(* Logix 5000 Rung export; software revision 16.03 *)

MODULES
   PDPMV1_240 : vendor None type None code None
   Local : vendor None type None code None
END_MODULES

TYPE PDPMV1_SetSlaveMode_Out :   // Mailbox Request
STRUCT
   GroupSelect : SINT;   // Range 01h to FFh (Bit Coded). This parameter determines which group to address. Refer to the user manual for examples
   SlaveAddress : SINT;   // Range 1 to 125; 127 (Multicast address).
   ControlCommand : PDPMV1_ControlCommand;   // This parameter specifies the command to send (Unsync/Sync and Unfreeze/Freeze).
END_STRUCT
END_TYPE

TYPE PDPMV1_AbortConnection_In :
STRUCT
   C_REF : INT;   // Connection reference that shall be terminated.
   ReasonCode : SINT;   // Indicates the reason for the abort request. Value is user-specific. Range 0...15
   Subnet : SINT;   // This parameter encodes information about the origin of the abort initiator. 0: No 1: Local 2: Remote 3...255: (reserved)
   ExtendedFaultInformation : INT;   // If ‘Fault Information’ equals 000Ah or 000Bh, additional information of the error can be found here. For more information,
   FaultInformation : INT;   // If ‘Invalid Other’ is returned in the Message Information word in the header of the response,
END_STRUCT
END_TYPE

TYPE PDPMV1_SetSlaveMode_In :   // Mailbox response
STRUCT
   GroupSelect : SINT;   // Range 01h to FFh (Bit Coded). This parameter determines which group to address. Refer to the user manual for examples
   SlaveAddress : SINT;   // Range 1 to 125; 127 (Multicast address).
   ControlCommand : PDPMV1_ControlCommand;   // This parameter specifies the command to send (Unsync/Sync and Unfreeze/Freeze).
   ExtendedFaultInfo : INT;   // If other than 0, refer to user manual for code information
   FaultInformation : INT;   // If other than 0, refer to user manual for code information
END_STRUCT
END_TYPE

TYPE PDPMV1_Class2AcyclicRead_Out :
STRUCT
   C_REF : INT;   // Connection reference that shall be terminated
   Index : SINT;   // Used in the slave for addressing of the desired data block. Range 0...254
   SlotNumber : SINT;   // Used in the slave for addressing of the desired data block. Range 0...254
   Length : INT;   // Number of bytes to write
END_STRUCT
END_TYPE

TYPE PDPMV1_Class1AcyclicRead :   // DPV1 acyclic read mailbox data structure
STRUCT
   Out : PDPMV1_Class1AcyclicRead_Out;   // Mailbox request
   In : PDPMV1_Class1AcyclicRead_In;   // Mailbox response
END_STRUCT
END_TYPE

TYPE PDPMV1_Class1AcyclicRead_In :   // DPV1 acyclic read mailbox response
STRUCT
   ByteCount : INT;   // Byte count data block
   SlotNumber : SINT;   // Used in the slave to address the desired data block.
   SlaveAddress : SINT;   // Destination of slave (1-125)
   Length : SINT;   // Specifies the number of bytes of the data block to read
   Index : SINT;   // Index block
   ErrorDecode : SINT;   // If other than 0, refer to user manual for code information
   ErrorCode2 : SINT;   // If other than 0, refer to user manual for code information
   ErrorCode1 : SINT;   // If other than 0, refer to user manual for code information
   ExtendedFaultInfo : SINT;   // If other than 0, refer to user manual for code information
   FaultInformation : SINT;   // If other than 0, refer to user manual for code information
   Data : SINT[244];   // Returned data [1...n] array
END_STRUCT
END_TYPE

TYPE PDPMV1_AbortConnection :
STRUCT
   Out : PDPMV1_AbortConnection_out;   // Mailbox Request
   In : PDPMV1_AbortConnection_In;   // Mailbox Response
END_STRUCT
END_TYPE

TYPE PDPMV1_SetSlaveMode :   // SetSlaveMode mailbox that allows the processor to change the slave mode to interrupt input or output data update
STRUCT
   Out : PDPMV1_SetSlaveMode_Out;   // Mailbox Request
   In : PDPMV1_SetSlaveMode_In;   // Mailbox Response
END_STRUCT
END_TYPE

TYPE PDPMV1_GetSlaveConfig :   // GetSlaveConfig mailobox to retrieve configuration data from specific PROFIBUS slaves
STRUCT
   Out : PDPMV1_GetSlaveConfig_Out;   // mailbox request
   In : PDPMV1_GetSlaveConfig_In;   // mailbox response
END_STRUCT
END_TYPE

TYPE PDPMV1_other_status :
STRUCT
   Cfg_file_error : INT;   // Bit0 = PDPMV1.CFG, Bit 1 = WATTCP.CFG, Bit 2 = PDPMV1.DDB, Bit3=PDPMV1.XML
   R_120 : INT;   // Not Used
   R_122 : INT;   // Not Used
   R_124 : INT;   // Not Used
   R_126 : INT;   // Not Used
   R_128 : INT;   // Not Used
   R_130 : INT;   // Not Used
   R_132 : INT;   // Not Used
   R_134 : INT;   // Not Used
   R_136 : INT;   // Not Used
   R_138 : INT;   // Not Used
   R_140 : INT;   // Not Used
   R_142 : INT;   // Not Used
   R_144 : INT;   // Not Used
   In_MB_queue : INT;   // Number of messages in the input mailbox queue
   Out_MB_queue : INT;   // Number of messages in the output mailbox queue
   Alarm_MB_queue : INT;   // Number of messages in the alarm mailbox queue
   Last_out_MB : INT;   // Number of messages in the output mailbox queue
   Cur_in_MB : INT;   // Number of messages currently in the input mailbox queue
   Cur_alarm_MB : INT;   // Number of messages currently in the alarm mailbox queue
END_STRUCT
END_TYPE

TYPE PDPMV1_Class1AcyclicWrite_In :   // DPV1 acyclic write mailbox response
STRUCT
   ByteCount : INT;   // Byte count data block
   SlotNumber : SINT;   // Used in the slave to address the desired data block.
   SlaveAddress : SINT;   // Destination of slave (1-125)
   Length : SINT;   // Specifies the number of bytes of the data block to read
   Index : SINT;   // Index block
   ErrorDecode : SINT;   // If other than 0, refer to user manual for code information
   ErrorCode2 : SINT;   // If other than 0, refer to user manual for code information
   ErrorCode1 : SINT;   // If other than 0, refer to user manual for code information
   ExtendedFaultInfo : SINT;   // If other than 0, refer to user manual for code information
   FaultInformation : SINT;   // If other than 0, refer to user manual for code information
   Data : SINT[244];   // Returned data [1...n] array
END_STRUCT
END_TYPE

TYPE PDPMV1_Class2AcyclicWrite_Out :   // DPV1 acyclic write mailbox request
STRUCT
   DataSize : INT;   // Object data size
   C_REF : INT;   // Connection reference that shall be terminated
   Index : SINT;   // Index block
   SlotNumber : SINT;   // Used in the slave to address the desired data block.
   Length : INT;   // Specifies the number of bytes of the data block to read
   Data : SINT[244];   // Data that should be written [1...n]
END_STRUCT
END_TYPE

TYPE PDPMV1_SetSlaveAddress_In :   // Mailbox response
STRUCT
   ByteCount : INT;   // Byte count data block
   NewSlaveAddress : SINT;   // Range 1 to 125, specifies the new address of the slave
   CurrentSlaveAddress : SINT;   // Range 1 to 125, specifies the current address of the slave
   SlaveIdentNumber : INT;   // Indent number for the slave
   No_add_Chg : INT;   // specifies whether it is allowed to change the slave address again later
   ErrorCode1_2 : INT;   // If other than 0, refer to user manual for code information
   ErrorCode3_4 : INT;   // If other than 0, refer to user manual for code information
   ReturnCode : INT;   // If other than 0, refer to user manual for code information
   FaultInformation : INT;   // If other than 0, refer to user manual for code information
   MessageDataByte : SINT[400];   // Message data byte array for user-specific data
END_STRUCT
END_TYPE

TYPE PDPMV1_SetSlaveAddress_Out :   // Mailbox request
STRUCT
   ByteCount : INT;   // Byte count data block
   NewSlaveAddress : SINT;   // Range 1 to 125, specifies the new address of the slave
   CurrentSlaveAddress : SINT;   // Range 1 to 125, specifies the current address of the slave
   SlaveIdentNumber : INT;   // Indent number for the slave
   No_add_Chg : INT;   // specifies whether it is allowed to change the slave address again later
   MessageDataByte : SINT[400];   // Message data byte array for user-specific data
END_STRUCT
END_TYPE

TYPE PDPMV1_backplane :   // This object stores variables used by the sample ladder for handshaking.
STRUCT
   Read : INT;   // Backplane read statistics
   Write : INT;   // Backplane write statistics
   Error : INT;   // Backplane error statistics
   LastRead : INT;   // Last read block index received from the module
   LastWrite : INT;   // Last write block index received from the module
   BlockIndex : INT;   // Block index of each copy of PROFIBUS input and output blocks
END_STRUCT
END_TYPE

TYPE PDPMV1_GetSlaveDiagnostics_In :   // GetSlaveDiagnostics mailbox response
STRUCT
   RequestType : SINT;   // Type of request. 0 to use module memory RAM or 1 for live PROFIBUS network.
   SlaveAddress : SINT;   // Destination of slave (Range 1-125)
   ExtendedFaultInfo : INT;   // If other than 0, refer to user manual for code information
   FaultInformation : INT;   // If other than 0, refer to user manual for code information
   StationStatus1_2 : INT;   // Status of station types 1 and 2
   StationStatus3_4 : INT;   // Status of station types 3 and 4
   IdentNumber : INT;   // Unique ID assigned by the PROFIBUS User Organization
   ExtendedDiagnosticData : INT[200];   // Slave user-specific data. Refer to actual slave documentation for info
END_STRUCT
END_TYPE

TYPE PDPMV1_ControlCommand :   // Option bits for SetSlaveMode mailbox
STRUCT
   Reserved1 : BOOL;   // Reserved
   Reserved2 : BOOL;   // Reserved
   Unfreeze_Input : BOOL;   // Freeze mode is concluded when initiated
   Freeze_Input : BOOL;   // Causes the addressed slave to assume freeze mode.
   Unsynchronize_Output : BOOL;   // Unsynchronized output data
   Synchronize_Output : BOOL;   // Synchronized output data
   Reserved3 : BOOL[32];   // Reserved
END_STRUCT
END_TYPE

TYPE PDPMV1_InitiateConnection_out :
STRUCT
   SlaveAddress : INT;   // Address of the slave to which a connection shall be established. Range: 0...126
   C_REF : INT;   // Connections references used to identify the connection later on. Range: 1-128
END_STRUCT
END_TYPE

TYPE PDPMV1_CRC :   // This object stores CRC values for both Profibus and the module.
STRUCT
   ProfibusCRC : DINT;   // Stores Profibus CRC32 values
   ModuleCRC : DINT;   // Stores Module CRC32 values
END_STRUCT
END_TYPE

TYPE PDPMV1_Fieldbus :   // Fieldbus status
STRUCT
   FB_Slave_Cfg_List : SINT[16];   // Bitmap structure containing PROFIBUS slave configuration (bit x = 1 means slave x is configured)
   FB_Slave_Data_xfer : SINT[16];   // Bitmap structure containing PROFIBUS slave data exchange status (bit x = 1 means slave x is transferring data to the module)
   FB_Slave_Diag : SINT[16];   // Bitmap structure containing PROFIBUS slave diagnostic info (bit x = 1 means slave x is reporting diagnostics)
   FB_Pad_Byte : SINT;   // Reserved
   FB_op_state : SINT;   // Operation state ( 00 = offline, 40 = stop, 80 = clear, C0= operate)
   FB_ident_MSB : SINT;   // Master identification code (most significant byte)
   FB_ident_LSB : SINT;   // Master identification code (least significant byte)
END_STRUCT
END_TYPE

TYPE PDPMV1_GetSlaveDiagnostics :   // GetSlaveDiagnostics mailbox to retrieve diagnostic information from specific PROFIBUS slaves
STRUCT
   Out : PDPMV1_GetSlaveDiagnostics_Out;   // Mailbox request
   In : PDPMV1_GetSlaveDiagnostics_In;   // Mailbox response
END_STRUCT
END_TYPE

TYPE PDPMV1_Class1AcyclicWrite_Out :   // DPV1 acyclic write mailbox request
STRUCT
   SlotNumber : SINT;   // Used in the slave to address the desired data block.
   SlaveAddress : SINT;   // Destination of slave (1-125)
   DataSize : INT;   // Object data size
   Length : SINT;   // Specifies the number of bytes of the data block to read
   Index : SINT;   // Index block
   Data : SINT[244];   // Data that should be written [1...n]
END_STRUCT
END_TYPE

TYPE PDPMV1_Module :   // Status data
STRUCT
   Mod_scan_count : INT;   // Incremented every module scan loop
   Mod_output_update : INT;   // Incremented at every output scan
   Mod_input_update : INT;   // Incremented at every input scan
   Mod_out_MB : INT;   // Incremented at every output mailbox processing
   Mod_in_MB : INT;   // Incremented at every intput mailbox processing
   Mod_alarm_ind : INT;   // Incremented at every alarm indication
   Mod_alarm_con : INT;   // Incremented at every alarm confirmation
   Reserved1 : INT;   // Reserved
   Reserved2 : INT;   // Reserved
END_STRUCT
END_TYPE

TYPE PDPMV1_Class1AcyclicRead_Out :   // DPV1 acyclic read mailbox request
STRUCT
   SlotNumber : SINT;   // Used in the slave to address the desired data block.
   SlaveAddress : SINT;   // Destination of slave (1-125)
   DataSize : INT;   // Object data size
   Length : SINT;   // Specifies the number of bytes of the data block to read
   Index : SINT;   // Index block
END_STRUCT
END_TYPE

TYPE PDPMV1_backplane2 :   // This object stores variables used by the sample ladder for handshaking.
STRUCT
   LastRead : INT;   // Last read block index received from the module
   LastWrite : INT;   // Last write block index received from the module
   BlockIndex : INT;   // Block index of each copy of PROFIBUS input and output blocks
END_STRUCT
END_TYPE

TYPE PDPMV1_Start_Stop_Slaves_In :   // Mailbox response
STRUCT
   AdditionalFaultInfo : INT;   // If other than 0, refer to user manual for code information
   FaultInformation : INT;   // If other than 0, refer to user manual for code information
   SlaveNumber : SINT[126];   // Slave number designation (1-125)
END_STRUCT
END_TYPE

TYPE PDPMV1_InitiateConnection :
STRUCT
   Out : PDPMV1_InitiateConnection_out;   // Mailbox Request
   In : PDPMV1_InitiateConnection_In;   // Mailbox response
END_STRUCT
END_TYPE

TYPE PDPMV1_Class2AcyclicRead_In :
STRUCT
   DataSize : INT;   // Byte count data block
   C_REF : INT;   // Connections references used to identify the connection later on. Range: 1-128
   Index : SINT;   // Index block
   SlotNumber : SINT;   // Used in the slave to address the desired data block.
   Length : INT;   // Specifies the number of bytes of the data block to read
   ErrorDecode : INT;   // If other than 0, refer to user manual for code information
   ErrorCode2 : SINT;   // If other than 0, refer to user manual for code information
   ErrorCode1 : SINT;   // If other than 0, refer to user manual for code information
   ExtendedFaultInfo : SINT;   // If other than 0, refer to user manual for code information
   FaultInformation : SINT;   // If other than 0, refer to user manual for code information
   Data : SINT[244];   // Returned data [1...n] array
END_STRUCT
END_TYPE

TYPE PDPMV1_Control :   // Control status
STRUCT
   serial_number : SINT[4];   // Module serial number
   version_MSB : SINT;   // Module version number (most significant byte)
   version_LSB : SINT;   // Module version number (least significant byte)
   mod_status_MSB : SINT;   // Module status (most significant byte)
   mod_status_LSB : SINT;   // Module status (least significant byte)
END_STRUCT
END_TYPE

TYPE PDPMV1_Command :   // This object contains the command bits that request mailbox messages from the module.
STRUCT
   StopMode : BOOL;   // Set the module to stop mode (PROFIBUS communication is interrupted in stop mode)
   OperateMode : BOOL;   // Set the module to operate mode (module only communicates through PROFIBUS)
   ClearMode : BOOL;   // Set the module to clear mode (outputs are disabled)
   SynchCRC : BOOL;   // CRC synchronization
   GetLiveList : BOOL;   // Request the Live List information from the module
   GetSlaveConfig : BOOL;   // Request configuration information from a slave
   SetSlaveMode : BOOL;   // Set the module to stop mode (PROFIBUS communication is interrupted in stop mode)
   GetSlaveDiagnostics : BOOL;   // Requests slave diagnostics from a slave
   SetSlaveAddress : BOOL;   // Change the slave's PROFIBUS address (only if slave supports this feature)
   StartSlaves : BOOL;   // Restarts PROFIBUS communication with one or more slaves after a "StopSlave" mailbox
   StopSlaves : BOOL;   // Stop PROFIBUS communication with one or more slaves
   Class1AcyclicRead : BOOL;   // Request the module to send acyclic read message to the slave
   Class1AcyclicWrite : BOOL;   // Request the module to send acyclic write message to slave
   InitiateConnection : BOOL;   // Request to establish connection with a V1 slave that can handle class 2 messages
   AbortConnection : BOOL;   // Request to Abort an already established connection with a V1 slave that can handle class 2 messages
   Class2AcyclicRead : BOOL;   // Request the module to send class 2 acyclic Read message to a V1 slave
   Class2AcyclicWrite : BOOL;   // Request the module to send class 2 acyclic Write message to a V1 slave
END_STRUCT
END_TYPE

TYPE PDPMV1_ModuleDef :   // Main module definition
STRUCT
   Output : SINT[1536];   // Output data
   Input : SINT[1536];   // Input data
   BP : PDPMV1_backplane2;   // Backplane status
   Status : PDPMV1_Status;   // Module status information
   MailboxCommand : PDPMV1_Command;   // Mailbox Command
   Mailbox : PDPMV1_Mailbox;   // Mailbox tags for optional applications
   CRC : PDPMV1_CRC_Struct;   // CRC status
   MailboxControl : PDPMV1_MBControl;   // Mailbox Control
   Util : PDPMV1_Util;   // Internal tags used for ladder logic processing. User applications should not overwrite any Util tags
END_STRUCT
END_TYPE

TYPE PDPMV1_GetSlaveConfig_Out :   // GetSlaveConfig mailbox request
STRUCT
   SlaveAddress : INT;   // Destination of slave (1-125)
END_STRUCT
END_TYPE

TYPE PDPMV1_GetSlaveDiagnostics_Out :   // GetSlaveDiagnostics mailbox request
STRUCT
   RequestType : SINT;   // Type of request. 0 to use module memory RAM or 1 for live PROFIBUS network.
   SlaveAddress : SINT;   // Destination of slave (Range 1-125)
END_STRUCT
END_TYPE

TYPE PDPMV1_Class1AcyclicWrite :   // DPV1 acyclic write mailbox data structure
STRUCT
   Out : PDPMV1_Class1AcyclicWrite_Out;   // Mailbox request
   In : PDPMV1_Class1AcyclicWrite_In;   // Mailbox response
END_STRUCT
END_TYPE

TYPE PDPMV1_InitiateConnection_In :   // This tag holds the response parameters after the user sends mailbox to initiate connection with V1 slave
STRUCT
   SizeofdatainBytes : INT;   // Size of data being read
   C_REF : INT;   // Connections references used to identify the connection later on. Range: 1-128
   MaxDataLength : SINT;   // The slave’s maximum data length in bytes (reported by the slave in DP Initiate.res).
   SlaveAddress : SINT;   // Address of the slave to which a connection shall be established. Range: 0...126
   MinmumSlaveTimeout : INT;   // The minimum slave timeout value supported by the slave (in multiples of 10ms).
   ErrorDecode : SINT;   // If ‘Fault Information’ equals 0010h, additional information according to the DPV1 specification
   ErrorCode2 : SINT;   // If ‘Fault Information’ equals 0010h, additional information according to the DPV1 specification
   ErrorCode1 : SINT;   // If ‘Fault Information’ equals 0010h, additional information according to the DPV1 specification
   ExtendedFaultInformation : INT;   // If ‘Fault Information’ equals 000Ah or 000Bh, additional information of the error can be found here. For more information, see
   FaultInformation : INT;   // If ‘Invalid Other’ is returned in the Message Information word in the header of the response, information about the fault
   SendTimeout : INT;   // Defines the control time (timebase 10ms) for the supervision of the connection between the slave and the master. Range 6...655
   FeatureSupported2 : SINT;   // (reserved for future use)
   FeatureSupported1 : SINT;   // Identifies the supported C2-service functionality as follows: b0: DPV1_RW. This bit is set if the services C2_Read and C2_Write
   ProfileFeatures2 : SINT;   // Identifies the supported service functionality regarding the used profile definition. The meaning of these registers are profil
   ProfileFeatures1 : SINT;   // Identifies the supported service functionality regarding the used profile definition. The meaning of these registers are profil
   ProfileIdentNumber : INT;   // This parameter identifies a unique profile definition. The Profile Ident Number is taken from the pool of Ident Numbers managed
   S_Length : SINT;   // This parameter specifies the length of the S_Address parameter (see table below). Default value is 02h.
   S_Type : SINT;   // This parameter indicates the presence of the optional Network/MAC address of the source. b0: 1: A Network/MAC address is presen
   D_Length : SINT;   // This value specifies the length of the D_Address parameter (see table below). Default value is 02h.
   D_Type : SINT;   // This parameter indicates the presence of the optional Network/MAC address of the destination. b0: 1: A Network/MAC address is p
   S_Address : INT;   // This field holds additional address information about the source. It’s structure depends on the settings in S_Type.
   D_Address : INT;   // This field holds additional address information about the destination. It’s structure depends on the settings in D_Type
END_STRUCT
END_TYPE

TYPE PDPMV1_Class2AcyclicWrite :   // DPV1 acyclic write mailbox data structure
STRUCT
   Out : PDPMV1_Class2AcyclicWrite_Out;   // Mailbox request
   In : PDPMV1_Class2AcyclicWrite_In;   // Mailbox response
END_STRUCT
END_TYPE

TYPE PDPMV1_GetLiveList :   // GetLiveList mailbox to retrieve the live list information from PROFIBUS network, informing the slaves that are communicating
STRUCT
   ReturnCode : SINT;   // Returned code about the nodes on the network
   FaultInfo : SINT;   // If other than 0, refer to user manual for code information
   Station : SINT[127];   // Station type contents.
END_STRUCT
END_TYPE

TYPE PDPMV1_AbortConnection_out :
STRUCT
   C_REF : INT;   // Connection reference that shall be terminated
   ReasonCode : SINT;   // Indicates the reason for the abort request. Value is user-specific. Range 0...15.
   Subnet : SINT;   // This parameter encodes information about the origin of the abort initiator. 0: No 1: Local 2: Remote
END_STRUCT
END_TYPE

TYPE PDPMV1_GetSlaveConfig_In :   // GetSlaveConfig mailbox response
STRUCT
   ByteCount : INT;   // Byte count data block
   WordCount : INT;   // Word count data block
   SlaveAddress : INT;   // Destination of slave (1-125)
   ErrorCode : INT[1];   // If other than 0, refer to user manual for code information
   ReturnCode : INT;   // If other than 0, refer to user manual for code information
   FaultInformation : INT;   // If other than 0, refer to user manual for code information
   Identifier : SINT[245];   // Configuration from a specific connected PROFIBUS slave
END_STRUCT
END_TYPE

TYPE PDPMV1_Util :
STRUCT
   ByteSwapUtil : INT;   // Used for byte swap logic
   TempInt : INT;   // Used for integer formatting
   UtilCount : INT;   // Used for util count range
END_STRUCT
END_TYPE

TYPE PDPMV1_CRC_Struct :   // Module CRC structures
STRUCT
   In : PDPMV1_CRC;   // Mailbox response
   Out : PDPMV1_CRC;   // Mailbox request
END_STRUCT
END_TYPE

TYPE PDPMV1_Class2AcyclicWrite_In :   // DPV1 acyclic write mailbox response
STRUCT
   ByteCount : INT;   // Byte count data block
   C_REF : INT;   // Connection reference that shall be Read
   Index : SINT;   // Index block
   SlotNumber : SINT;   // Used in the slave to address the desired data block.
   Length : SINT;   // Specifies the number of bytes of the data block to read
   ErrorDecode : SINT;   // If other than 0, refer to user manual for code information
   ErrorCode2 : SINT;   // If other than 0, refer to user manual for code information
   ErrorCode1 : SINT;   // If other than 0, refer to user manual for code information
   ExtendedFaultInfo : SINT;   // If other than 0, refer to user manual for code information
   FaultInformation : SINT;   // If other than 0, refer to user manual for code information
   Data : SINT[244];   // Returned data [1...n] array
END_STRUCT
END_TYPE

TYPE PDPMV1_MBControl :   // PDPMV1 MBControl status.
STRUCT
   Out_MB_index : INT;   // Reserved
   In_MB_index : INT;   // Reserved
   Alarm_MB_index : INT;   // Reserved
   In_Last_Out_MB : INT;   // Last out mailbox message ID processed from output image
   In_Last_In_MB : INT;   // Current in mailbox control index
   In_Last_Alarm_MB : INT;   // Current alarm control index
   Out_Last_Out_MB : INT;   // Reserved
   Out_Last_In_MB : INT;   // Reserved
   Out_Last_Alarm_MB : INT;   // Reserved
END_STRUCT
END_TYPE

TYPE PDPMV1_Start_Stop_Slaves_Out :   // Mailbox request
STRUCT
   SlaveNumber : SINT[126];   // Slave number designation (1-125)
END_STRUCT
END_TYPE

TYPE PDPMV1_Mailbox :   // Stores all mailbox request and response registers
STRUCT
   GetLiveList : PDPMV1_GetLiveList;   // Gets information from all nodes on the network
   GetSlaveConfig : PDPMV1_GetSlaveConfig;   // Get slave configuration
   SetSlaveMode : PDPMV1_SetSlaveMode;   // Send special control command to one or several slaves (Sync/Freeze)
   GetSlaveDiagnostics : PDPMV1_GetSlaveDiagnostics;   // Get diagnostic information from a slave
   SetSlaveAddress : PDPMV1_SetSlaveAddress;   // Set node address of a slave (if supported by the slave)
   StartStopSlaves : PDPMV1_Start_Stop_Slaves;   // Start/Stop slaves dynamically
   Class1AcyclicRead : PDPMV1_Class1AcyclicRead;   // Initiates a DPV1 class 1 acyclic read request.
   Class1AcyclicWrite : PDPMV1_Class1AcyclicWrite;   // Initiates a DPV1 class 1 acyclic write request.
   Alarm : PDPMV1_Alarm;   // Alarm message transferred by a slave to the master
   InitiateConnection : PDPMV1_InitiateConnection;   // mailbox form used to initiate connection with v1 slave before sending class2 messages.
   AbortConnection : PDPMV1_AbortConnection;   // mailbox form used to abort an already established connection with v1 slave before sending class2 messages.
   Class2AcyclicRead : PDPMV1_Class2AcyclicRead;   // mailbox form used to send a class 2 messages to read acyclic data
   Class2AcyclicWrite : PDPMV1_Class2AcyclicWrite;
END_STRUCT
END_TYPE

TYPE PDPMV1_Start_Stop_Slaves :   // Start/Stop Slaves mailbox allows the processor to restart or hault slave communication.
STRUCT
   Out : PDPMV1_Start_Stop_Slaves_Out;   // Mailbox Request
   In : PDPMV1_Start_Stop_Slaves_In;   // Mailbox Response
END_STRUCT
END_TYPE

TYPE PDPMV1_Alarm :   // DPV1 alarm data received by the module
STRUCT
   ByteCount : INT;   // Byte count data block
   SlotNumber : SINT;   // Used in the slave to address the desired data block. Range 0-254
   SlaveAddress : SINT;   // Destination of slave (1-125)
   AlarmSpecAck : SINT;   // Additional alarm information
   SeqNumber : SINT;   // Unique ID number of the alarm. Range 0-31.
   ExtDiag : SINT;   // Extended Diagnostic Flag (FFh - flag set and 00h - flag cleared).
   AlarmType : SINT;   // Identifies alarm type. Range is from 1 to 6, 32 to 126.
   FaultInformation : SINT;   // If other than 0, refer to user manual for code information
   Data : SINT[500];   // Returned data [1...n] array with additional manf. spec alarm info.
END_STRUCT
END_TYPE

TYPE PDPMV1_SetSlaveAddress :   // SetSlaveAddress mailbox that allows the module to dynamically change a PRIDUBUS address (only for slaves that supports it)
STRUCT
   Out : PDPMV1_SetSlaveAddress_Out;   // Mailbox request
   In : PDPMV1_SetSlaveAddress_In;   // Mailbox response
END_STRUCT
END_TYPE

TYPE PDPMV1_Class2AcyclicRead :
STRUCT
   Out : PDPMV1_Class2AcyclicRead_Out;   // Mailbox request
   In : PDPMV1_Class2AcyclicRead_In;   // Mailbox response
END_STRUCT
END_TYPE

TYPE PDPMV1_Status :   // Status block 0 or -1 for the MVI56-PDPMV1 module
STRUCT
   Pattern : SINT[12];   // Module indentification code
   Input_Size : INT;   // Input data size
   Output_Size : INT;   // Output data size
   Reserved_16 : INT;   // Reserved
   Reserved_18 : INT;   // Reserved
   Reserved_20 : INT;   // Reserved
   Input_Swap : SINT;   // User configured flag to indicate if input data is swapped before placing in the input image of the controller
   Output_Swap : SINT;   // User configured flag to indicate if output data is swapped before placing in the output image of the controller
   Module_Major_Ver : SINT;   // Module software major version number
   Module_Minor_Ver : SINT;   // Module software minor version number
   Fieldbus : PDPMV1_Fieldbus;   // PROFIBUS network status information
   Control : PDPMV1_Control;   // Module information
   Profibus_CRC32 : DINT;   // Profibus CRC32 value
   Module_CRC32 : DINT;   // Module CRC32 value
   Module : PDPMV1_Module;   // General module status to monitor data, mailbox and alarm exchange between the processor and the module
   Backplane : PDPMV1_backplane;   // Backplane status information
   Other : PDPMV1_other_status;   // General mailbox and cfg error information
END_STRUCT
END_TYPE

ADD_ON_INSTRUCTION AOI69PDPMV1_240   (* revision 1.4, vendor ProSoft Technology Inc. *)
// Add-On - MVI69-PDPMV1(Block size 240).
// Revision note:
// v1.4 - Added support for class 2 messages that was supported in a specific  V1 slaves.
VAR_IN_OUT
   Connection_Input : INT[242]; {required}   // Connection Input to be associated to the MVI69PDPMV1 Input Array
   Connection_Output : INT[241]; {required}   // Connection Output to be associated to the MVI69-PDPMV1 Output Array
   MVI69PDPMV1 : PDPMV1_ModuleDef; {required}
END_VAR

ROUTINE Logic   (* ladder *)
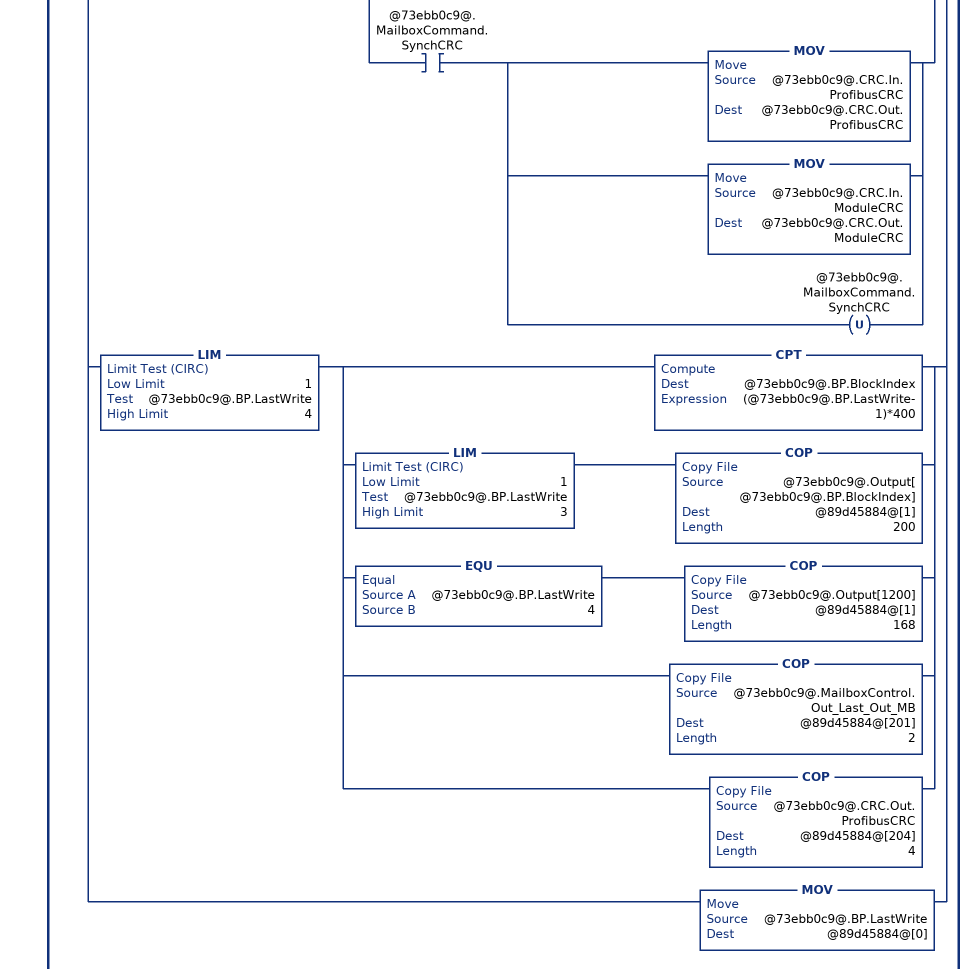
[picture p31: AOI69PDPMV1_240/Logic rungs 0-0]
   // This rung is used to verify if the module has sent a new input block to the processor. The trigger is when the input image offset 0 (Read Block ID) is different than the last one processed by the processor
   0: NEQ(@8034a877@[0],@73ebb0c9@.BP.LastRead)[MOV(@8034a877@[0],@73ebb0c9@.BP.LastRead) ,[EQU(@73ebb0c9@.BP.LastRead,-1) ,EQU(@73ebb0c9@.BP.LastRead,0) ] [COP(@8034a877@[2],@73ebb0c9@.Status.Pattern[0],20) ,COP(@8034a877@[13],@73ebb0c9@.Status.Input_Swap,4) ,COP(@8034a877@[15],@73ebb0c9@.Status.Fieldbus.FB_Slave_Cfg_List[0],52) ,COP(@8034a877@[41],@73ebb0c9@.Status.Control.serial_number[0],8) ,COP(@8034a877@[45],@73ebb0c9@.Status.Profibus_CRC32,2) ,COP(@8034a877@[49],@73ebb0c9@.Status.Module.Mod_scan_count,9) ,COP(@8034a877@[58],@73ebb0c9@.Status.Backplane.Read,3) ,COP(@8034a877@[61],@73ebb0c9@.Status.Other.Cfg_file_error,20) ] ,LIM(1,@73ebb0c9@.BP.LastRead,4) [LIM(1,@73ebb0c9@.BP.LastRead,3) [CPT(@73ebb0c9@.BP.BlockIndex,(@73ebb0c9@.BP.LastRead-1)*400) ,COP(@8034a877@[2],@73ebb0c9@.Input[@73ebb0c9@.BP.BlockIndex],400) ] ,EQU(@73ebb0c9@.BP.LastRead,4) COP(@8034a877@[2],@73ebb0c9@.Input[1200],336) ,COP(@8034a877@[202],@73ebb0c9@.MailboxControl.In_Last_Out_MB,2) ,COP(@8034a877@[206],@73ebb0c9@.CRC.In.ProfibusCRC,2) ] ,LIM(100,@73ebb0c9@.BP.LastRead,109) [LIM(0,@8034a877@[2],2) [OTU(@73ebb0c9@.MailboxCommand.StopMode) ,OTU(@73ebb0c9@.MailboxCommand.OperateMode) ,OTU(@73ebb0c9@.MailboxCommand.ClearMode) ,OTU(@73ebb0c9@.MailboxCommand.SynchCRC) ,OTU(@73ebb0c9@.MailboxCommand.GetLiveList) ,OTU(@73ebb0c9@.MailboxCommand.GetSlaveConfig) ,OTU(@73ebb0c9@.MailboxCommand.SetSlaveMode) ,OTU(@73ebb0c9@.MailboxCommand.GetSlaveDiagnostics) ,OTU(@73ebb0c9@.MailboxCommand.SetSlaveAddress) ,OTU(@73ebb0c9@.MailboxCommand.Class1AcyclicRead) ,OTU(@73ebb0c9@.MailboxCommand.Class1AcyclicWrite) ,OTU(@73ebb0c9@.MailboxCommand.StartSlaves) ,OTU(@73ebb0c9@.MailboxCommand.StopSlaves) ,OTU(@73ebb0c9@.MailboxCommand.InitiateConnection) ,OTU(@73ebb0c9@.MailboxCommand.AbortConnection) ,OTU(@73ebb0c9@.MailboxCommand.Class2AcyclicRead) ,OTU(@73ebb0c9@.MailboxCommand.Class2AcyclicWrite) ] ,EQU(@8034a877@[4],24) COP(@8034a877@[18],@73ebb0c9@.Mailbox.GetLiveList.Station[0],127) ,EQU(@8034a877@[4],3) [COP(@8034a877@[10],@73ebb0c9@.Mailbox.SetSlaveMode.In.GroupSelect,2) ,MOV(@8034a877@[11],@73ebb0c9@.Util.TempInt) ,SWPB(@73ebb0c9@.Util.TempInt,REVERSE,@73ebb0c9@.Util.ByteSwapUtil) ,COP(@73ebb0c9@.Util.ByteSwapUtil,@73ebb0c9@.Mailbox.SetSlaveMode.In.ControlCommand,1) ,MOV(@8034a877@[16],@73ebb0c9@.Mailbox.SetSlaveMode.In.ExtendedFaultInfo) ,MOV(@8034a877@[17],@73ebb0c9@.Mailbox.SetSlaveMode.In.FaultInformation) ] ,EQU(@8034a877@[4],4) [MOV(@8034a877@[5],@73ebb0c9@.Util.UtilCount) ,COP(@8034a877@[10],@73ebb0c9@.Mailbox.GetSlaveDiagnostics.In.RequestType,2) ,MOV(@8034a877@[16],@73ebb0c9@.Mailbox.GetSlaveDiagnostics.In.ExtendedFaultInfo) ,MOV(@8034a877@[17],@73ebb0c9@.Mailbox.GetSlaveDiagnostics.In.FaultInformation) ,MOV(@8034a877@[18],@73ebb0c9@.Mailbox.GetSlaveDiagnostics.In.StationStatus1_2) ,MOV(@8034a877@[19],@73ebb0c9@.Mailbox.GetSlaveDiagnostics.In.StationStatus3_4) ,MOV(@8034a877@[20],@73ebb0c9@.Mailbox.GetSlaveDiagnostics.In.IdentNumber) ,COP(@8034a877@[21],@73ebb0c9@.Mailbox.GetSlaveDiagnostics.In.ExtendedDiagnosticData[0],200) ] ,EQU(@8034a877@[4],5) [MOV(@8034a877@[5],@73ebb0c9@.Mailbox.GetSlaveConfig.In.ByteCount) ,MOV(@8034a877@[10],@73ebb0c9@.Util.ByteSwapUtil) ,SWPB(@73ebb0c9@.Util.ByteSwapUtil,REVERSE,@73ebb0c9@.Mailbox.GetSlaveConfig.In.SlaveAddress) ,COP(@8034a877@[14],@73ebb0c9@.Mailbox.GetSlaveConfig.In.ErrorCode[0],2) ,MOV(@8034a877@[16],@73ebb0c9@.Mailbox.GetSlaveConfig.In.ReturnCode) ,MOV(@8034a877@[17],@73ebb0c9@.Mailbox.GetSlaveConfig.In.FaultInformation) ,COP(@8034a877@[18],@73ebb0c9@.Mailbox.GetSlaveConfig.In.Identifier[0],@73ebb0c9@.Mailbox.GetSlaveConfig.In.ByteCount) ] ,EQU(@8034a877@[4],6) [MOV(@8034a877@[5],@73ebb0c9@.Mailbox.SetSlaveAddress.In.ByteCount) ,COP(@8034a877@[10],@73ebb0c9@.Mailbox.SetSlaveAddress.In.NewSlaveAddress,2) ,MOV(@8034a877@[11],@73ebb0c9@.Mailbox.SetSlaveAddress.In.SlaveIdentNumber) ,MOV(@8034a877@[12],@73ebb0c9@.Util.ByteSwapUtil) ,SWPB(@73ebb0c9@.Util.ByteSwapUtil,REVERSE,@73ebb0c9@.Mailbox.SetSlaveAddress.In.No_add_Chg) ,MOV(@8034a877@[14],@73ebb0c9@.Mailbox.SetSlaveAddress.In.ErrorCode1_2) ,MOV(@8034a877@[15],@73ebb0c9@.Mailbox.SetSlaveAddress.In.ErrorCode3_4) ,MOV(@8034a877@[16],@73ebb0c9@.Mailbox.SetSlaveAddress.In.ReturnCode) ,MOV(@8034a877@[17],@73ebb0c9@.Mailbox.SetSlaveAddress.In.FaultInformation) ,COP(@8034a877@[18],@73ebb0c9@.Mailbox.SetSlaveAddress.In.MessageDataByte[0],@73ebb0c9@.Mailbox.SetSlaveAddress.In.ByteCount) ] ,LIM(11,@8034a877@[4],12) [MOV(@8034a877@[16],@73ebb0c9@.Mailbox.StartStopSlaves.In.AdditionalFaultInfo) ,MOV(@8034a877@[17],@73ebb0c9@.Mailbox.StartStopSlaves.In.FaultInformation) ,COP(@8034a877@[18],@73ebb0c9@.Mailbox.StartStopSlaves.In.SlaveNumber[0],127) ] ,EQU(@8034a877@[4],32) [MOV(@8034a877@[5],@73ebb0c9@.Mailbox.Class1AcyclicRead.In.ByteCount) ,COP(@8034a877@[10],@73ebb0c9@.Mailbox.Class1AcyclicRead.In.SlotNumber,2) ,COP(@8034a877@[11],@73ebb0c9@.Mailbox.Class1AcyclicRead.In.Length,2) ,COP(@8034a877@[14],@73ebb0c9@.Mailbox.Class1AcyclicRead.In.ErrorDecode,1) ,COP(@8034a877@[15],@73ebb0c9@.Mailbox.Class1AcyclicRead.In.ErrorCode2,2) ,MOV(@8034a877@[16],@73ebb0c9@.Mailbox.Class1AcyclicRead.In.ExtendedFaultInfo) ,MOV(@8034a877@[17],@73ebb0c9@.Mailbox.Class1AcyclicRead.In.FaultInformation) ,COP(@8034a877@[18],@73ebb0c9@.Mailbox.Class1AcyclicRead.In.Data[0],@73ebb0c9@.Mailbox.Class1AcyclicRead.In.ByteCount) ] ,EQU(@8034a877@[4],33) [MOV(@8034a877@[5],@73ebb0c9@.Mailbox.Class1AcyclicWrite.In.ByteCount) ,COP(@8034a877@[10],@73ebb0c9@.Mailbox.Class1AcyclicWrite.In.SlotNumber,2) ,COP(@8034a877@[11],@73ebb0c9@.Mailbox.Class1AcyclicWrite.In.Length,2) ,COP(@8034a877@[14],@73ebb0c9@.Mailbox.Class1AcyclicWrite.In.ErrorDecode,1) ,COP(@8034a877@[15],@73ebb0c9@.Mailbox.Class1AcyclicWrite.In.ErrorCode2,2) ,MOV(@8034a877@[16],@73ebb0c9@.Mailbox.Class1AcyclicWrite.In.ExtendedFaultInfo) ,MOV(@8034a877@[17],@73ebb0c9@.Mailbox.Class1AcyclicWrite.In.FaultInformation) ,COP(@8034a877@[18],@73ebb0c9@.Mailbox.Class1AcyclicWrite.In.Data[0],@73ebb0c9@.Mailbox.Class1AcyclicWrite.In.ByteCount) ] ,EQU(@8034a877@[4],37) [MOV(@8034a877@[5],@73ebb0c9@.Mailbox.InitiateConnection.In.SizeofdatainBytes) ,MOV(@8034a877@[10],@73ebb0c9@.Mailbox.InitiateConnection.In.C_REF) ,COP(@8034a877@[11],@73ebb0c9@.Mailbox.InitiateConnection.In.MaxDataLength,2) ,MOV(@8034a877@[12],@73ebb0c9@.Mailbox.InitiateConnection.In.MinmumSlaveTimeout) ,COP(@8034a877@[14],@73ebb0c9@.Mailbox.InitiateConnection.In.ErrorDecode,1) ,COP(@8034a877@[15],@73ebb0c9@.Mailbox.InitiateConnection.In.ErrorCode2,2) ,MOV(@8034a877@[16],@73ebb0c9@.Mailbox.InitiateConnection.In.ExtendedFaultInformation) ,MOV(@8034a877@[17],@73ebb0c9@.Mailbox.InitiateConnection.In.FaultInformation) ,MOV(@8034a877@[18],@73ebb0c9@.Mailbox.InitiateConnection.In.SendTimeout) ,COP(@8034a877@[19],@73ebb0c9@.Mailbox.InitiateConnection.In.FeatureSupported2,2) ,COP(@8034a877@[20],@73ebb0c9@.Mailbox.InitiateConnection.In.ProfileFeatures2,2) ,MOV(@8034a877@[21],@73ebb0c9@.Mailbox.InitiateConnection.In.ProfileIdentNumber) ,COP(@8034a877@[22],@73ebb0c9@.Mailbox.InitiateConnection.In.S_Length,2) ,COP(@8034a877@[23],@73ebb0c9@.Mailbox.InitiateConnection.In.D_Length,2) ,MOV(@8034a877@[24],@73ebb0c9@.Mailbox.InitiateConnection.In.S_Address) ,MOV(@8034a877@[25],@73ebb0c9@.Mailbox.InitiateConnection.In.D_Address) ] ,EQU(@8034a877@[4],38) [MOV(@8034a877@[10],@73ebb0c9@.Mailbox.AbortConnection.In.C_REF) ,COP(@8034a877@[11],@73ebb0c9@.Mailbox.AbortConnection.In.ReasonCode,2) ,MOV(@8034a877@[16],@73ebb0c9@.Mailbox.AbortConnection.In.ExtendedFaultInformation) ,MOV(@8034a877@[17],@73ebb0c9@.Mailbox.AbortConnection.In.FaultInformation) ] ,EQU(@8034a877@[4],39) [MOV(@8034a877@[5],@73ebb0c9@.Mailbox.Class2AcyclicRead.In.DataSize) ,MOV(@8034a877@[10],@73ebb0c9@.Mailbox.Class2AcyclicRead.In.C_REF) ,COP(@8034a877@[11],@73ebb0c9@.Mailbox.Class2AcyclicRead.In.Index,2) ,COP(@8034a877@[12],@73ebb0c9@.Mailbox.Class2AcyclicRead.In.Length,1) ,COP(@8034a877@[14],@73ebb0c9@.Mailbox.Class2AcyclicRead.In.ErrorDecode,1) ,COP(@8034a877@[15],@73ebb0c9@.Mailbox.Class2AcyclicRead.In.ErrorCode2,2) ,MOV(@8034a877@[16],@73ebb0c9@.Mailbox.Class2AcyclicRead.In.ExtendedFaultInfo) ,MOV(@8034a877@[17],@73ebb0c9@.Mailbox.Class2AcyclicRead.In.FaultInformation) ,COP(@8034a877@[18],@73ebb0c9@.Mailbox.Class2AcyclicRead.In.Data[0],244) ] ,EQU(@8034a877@[4],40) [MOV(@8034a877@[5],@73ebb0c9@.Mailbox.Class2AcyclicWrite.In.ByteCount) ,MOV(@8034a877@[10],@73ebb0c9@.Mailbox.Class2AcyclicWrite.In.C_REF) ,COP(@8034a877@[11],@73ebb0c9@.Mailbox.Class2AcyclicWrite.In.Index,2) ,COP(@8034a877@[12],@73ebb0c9@.Mailbox.Class2AcyclicWrite.In.Length,1) ,COP(@8034a877@[14],@73ebb0c9@.Mailbox.Class2AcyclicWrite.In.ErrorDecode,1) ,COP(@8034a877@[15],@73ebb0c9@.Mailbox.Class2AcyclicWrite.In.ErrorCode2,2) ,MOV(@8034a877@[16],@73ebb0c9@.Mailbox.Class2AcyclicWrite.In.ExtendedFaultInfo) ,MOV(@8034a877@[17],@73ebb0c9@.Mailbox.Class2AcyclicWrite.In.FaultInformation) ,COP(@8034a877@[18],@73ebb0c9@.Mailbox.Class2AcyclicWrite.In.Data[0],244) ] ] ,LIM(200,@73ebb0c9@.BP.LastRead,209) [MOV(@8034a877@[5],@73ebb0c9@.Mailbox.Alarm.ByteCount) ,COP(@8034a877@[10],@73ebb0c9@.Mailbox.Alarm.SlotNumber,2) ,COP(@8034a877@[11],@73ebb0c9@.Mailbox.Alarm.AlarmSpecAck,2) ,COP(@8034a877@[12],@73ebb0c9@.Mailbox.Alarm.ExtDiag,2) ,MOV(@8034a877@[17],@73ebb0c9@.Mailbox.Alarm.FaultInformation) ,COP(@8034a877@[18],@73ebb0c9@.Mailbox.Alarm.Data[0],@73ebb0c9@.Mailbox.Alarm.ByteCount) ] ,EQU(@8034a877@[0],@73ebb0c9@.BP.LastRead) [MOV(@8034a877@[1],@73ebb0c9@.BP.LastWrite) ,XIC(@73ebb0c9@.MailboxCommand.StopMode) [MOV(100,@73ebb0c9@.BP.LastWrite) ,MOV(2,@89d45884@[1]) ,MOV(16386,@89d45884@[2]) ,MOV(2,@89d45884@[3]) ,MOV(0,@89d45884@[4]) ,MOV(1,@89d45884@[5]) ,MOV(1,@89d45884@[6]) ,MOV(0,@89d45884@[7]) ,MOV(0,@89d45884@[8]) ,MOV(16384,@89d45884@[9]) ] ,XIC(@73ebb0c9@.MailboxCommand.OperateMode) [MOV(101,@73ebb0c9@.BP.LastWrite) ,MOV(1,@89d45884@[1]) ,MOV(16386,@89d45884@[2]) ,MOV(2,@89d45884@[3]) ,MOV(0,@89d45884@[4]) ,MOV(1,@89d45884@[5]) ,MOV(1,@89d45884@[6]) ,MOV(0,@89d45884@[7]) ,MOV(0,@89d45884@[8]) ,MOV(-16384,@89d45884@[9]) ] ,XIC(@73ebb0c9@.MailboxCommand.ClearMode) [MOV(102,@73ebb0c9@.BP.LastWrite) ,MOV(3,@89d45884@[1]) ,MOV(16386,@89d45884@[2]) ,MOV(2,@89d45884@[3]) ,MOV(0,@89d45884@[4]) ,MOV(1,@89d45884@[5]) ,MOV(1,@89d45884@[6]) ,MOV(0,@89d45884@[7]) ,MOV(0,@89d45884@[8]) ,MOV(-32768,@89d45884@[9]) ] ,XIC(@73ebb0c9@.MailboxCommand.GetLiveList) [MOV(103,@73ebb0c9@.BP.LastWrite) ,MOV(4,@89d45884@[1]) ,MOV(16386,@89d45884@[2]) ,MOV(24,@89d45884@[3]) ,MOV(0,@89d45884@[4]) ,MOV(1,@89d45884@[5]) ,MOV(1,@89d45884@[6]) ,MOV(0,@89d45884@[7]) ,MOV(0,@89d45884@[8]) ] ,XIC(@73ebb0c9@.MailboxCommand.GetSlaveConfig) [MOV(104,@73ebb0c9@.BP.LastWrite) ,MOV(5,@89d45884@[1]) ,MOV(16386,@89d45884@[2]) ,MOV(5,@89d45884@[3]) ,MOV(0,@89d45884@[4]) ,MOV(1,@89d45884@[5]) ,MOV(1,@89d45884@[6]) ,MOV(0,@89d45884@[7]) ,MOV(0,@89d45884@[8]) ,SWPB(@73ebb0c9@.Mailbox.GetSlaveConfig.Out.SlaveAddress,REVERSE,@73ebb0c9@.Util.ByteSwapUtil) ,MOV(@73ebb0c9@.Util.ByteSwapUtil,@89d45884@[9]) ] ,XIC(@73ebb0c9@.MailboxCommand.SetSlaveMode) [MOV(105,@73ebb0c9@.BP.LastWrite) ,MOV(6,@89d45884@[1]) ,MOV(16386,@89d45884@[2]) ,MOV(3,@89d45884@[3]) ,MOV(0,@89d45884@[4]) ,MOV(1,@89d45884@[5]) ,MOV(1,@89d45884@[6]) ,MOV(0,@89d45884@[7]) ,MOV(0,@89d45884@[8]) ,COP(@73ebb0c9@.Mailbox.SetSlaveMode.Out.GroupSelect,@89d45884@[9],1) ,COP(@73ebb0c9@.Mailbox.SetSlaveMode.Out.ControlCommand,@73ebb0c9@.Util.TempInt,1) ,SWPB(@73ebb0c9@.Util.TempInt,REVERSE,@73ebb0c9@.Util.ByteSwapUtil) ,MOV(@73ebb0c9@.Util.ByteSwapUtil,@89d45884@[10]) ] ,XIC(@73ebb0c9@.MailboxCommand.GetSlaveDiagnostics) [MOV(106,@73ebb0c9@.BP.LastWrite) ,MOV(7,@89d45884@[1]) ,MOV(16386,@89d45884@[2]) ,MOV(4,@89d45884@[3]) ,MOV(0,@89d45884@[4]) ,MOV(1,@89d45884@[5]) ,MOV(1,@89d45884@[6]) ,MOV(0,@89d45884@[7]) ,MOV(0,@89d45884@[8]) ,COP(@73ebb0c9@.Mailbox.GetSlaveDiagnostics.Out.RequestType,@89d45884@[9],1) ] ,XIC(@73ebb0c9@.MailboxCommand.SetSlaveAddress) [MOV(107,@73ebb0c9@.BP.LastWrite) ,MOV(8,@89d45884@[1]) ,MOV(16386,@89d45884@[2]) ,MOV(6,@89d45884@[3]) ,MOV(@73ebb0c9@.Mailbox.SetSlaveAddress.Out.ByteCount,@89d45884@[4]) ,MOV(1,@89d45884@[5]) ,MOV(1,@89d45884@[6]) ,MOV(0,@89d45884@[7]) ,MOV(0,@89d45884@[8]) ,COP(@73ebb0c9@.Mailbox.SetSlaveAddress.Out.NewSlaveAddress,@89d45884@[9],1) ,MOV(@73ebb0c9@.Mailbox.SetSlaveAddress.Out.SlaveIdentNumber,@89d45884@[10]) ,SWPB(@73ebb0c9@.Mailbox.SetSlaveAddress.Out.No_add_Chg,REVERSE,@73ebb0c9@.Util.ByteSwapUtil) ,MOV(@73ebb0c9@.Util.ByteSwapUtil,@89d45884@[11]) ,COP(@73ebb0c9@.Mailbox.SetSlaveAddress.In.MessageDataByte[0],@89d45884@[17],100) ] ,XIC(@73ebb0c9@.MailboxCommand.StartSlaves) [MOV(105,@73ebb0c9@.BP.LastWrite) ,MOV(16,@89d45884@[1]) ,MOV(16386,@89d45884@[2]) ,MOV(11,@89d45884@[3]) ,MOV(126,@89d45884@[4]) ,MOV(1,@89d45884@[5]) ,MOV(1,@89d45884@[6]) ,MOV(0,@89d45884@[7]) ,MOV(0,@89d45884@[8]) ,MOV(0,@89d45884@[9]) ,MOV(0,@89d45884@[10]) ,MOV(0,@89d45884@[11]) ,MOV(0,@89d45884@[12]) ,MOV(0,@89d45884@[13]) ,MOV(0,@89d45884@[14]) ,MOV(0,@89d45884@[15]) ,MOV(0,@89d45884@[16]) ,COP(@73ebb0c9@.Mailbox.StartStopSlaves.Out.SlaveNumber[0],@89d45884@[17],126) ] ,XIC(@73ebb0c9@.MailboxCommand.StopSlaves) [MOV(106,@73ebb0c9@.BP.LastWrite) ,MOV(17,@89d45884@[1]) ,MOV(16386,@89d45884@[2]) ,MOV(12,@89d45884@[3]) ,MOV(126,@89d45884@[4]) ,MOV(1,@89d45884@[5]) ,MOV(1,@89d45884@[6]) ,MOV(0,@89d45884@[7]) ,MOV(0,@89d45884@[8]) ,MOV(0,@89d45884@[9]) ,MOV(0,@89d45884@[10]) ,MOV(0,@89d45884@[11]) ,MOV(0,@89d45884@[12]) ,MOV(0,@89d45884@[13]) ,MOV(0,@89d45884@[14]) ,MOV(0,@89d45884@[15]) ,MOV(0,@89d45884@[16]) ,COP(@73ebb0c9@.Mailbox.StartStopSlaves.Out.SlaveNumber[0],@89d45884@[17],126) ] ,XIC(@73ebb0c9@.MailboxCommand.Class1AcyclicRead) [MOV(108,@73ebb0c9@.BP.LastWrite) ,MOV(9,@89d45884@[1]) ,MOV(16386,@89d45884@[2]) ,MOV(32,@89d45884@[3]) ,COP(@73ebb0c9@.Mailbox.Class1AcyclicRead.Out.DataSize,@73ebb0c9@.Mailbox.Class1AcyclicRead.Out.Length,1) ,MOV(0,@89d45884@[4]) ,MOV(1,@89d45884@[5]) ,MOV(1,@89d45884@[6]) ,MOV(0,@89d45884@[7]) ,MOV(0,@89d45884@[8]) ,COP(@73ebb0c9@.Mailbox.Class1AcyclicRead.Out.SlotNumber,@89d45884@[9],1) ,COP(@73ebb0c9@.Mailbox.Class1AcyclicRead.Out.Length,@89d45884@[10],1) ] ,XIC(@73ebb0c9@.MailboxCommand.Class1AcyclicWrite) [MOV(100,@73ebb0c9@.BP.LastWrite) ,MOV(9,@89d45884@[1]) ,MOV(16386,@89d45884@[2]) ,MOV(33,@89d45884@[3]) ,COP(@73ebb0c9@.Mailbox.Class1AcyclicWrite.Out.DataSize,@73ebb0c9@.Mailbox.Class1AcyclicWrite.Out.Length,1) ,MOV(@73ebb0c9@.Mailbox.Class1AcyclicWrite.Out.DataSize,@89d45884@[4]) ,MOV(1,@89d45884@[5]) ,MOV(1,@89d45884@[6]) ,MOV(0,@89d45884@[7]) ,MOV(0,@89d45884@[8]) ,COP(@73ebb0c9@.Mailbox.Class1AcyclicWrite.Out.SlotNumber,@89d45884@[9],1) ,COP(@73ebb0c9@.Mailbox.Class1AcyclicWrite.Out.Length,@89d45884@[10],1) ,COP(@73ebb0c9@.Mailbox.Class1AcyclicWrite.Out.Data[0],@89d45884@[17],@73ebb0c9@.Mailbox.Class1AcyclicWrite.Out.Length) ] ,XIC(@73ebb0c9@.MailboxCommand.InitiateConnection) [MOV(100,@73ebb0c9@.BP.LastWrite) ,MOV(10,@89d45884@[1]) ,MOV(16386,@89d45884@[2]) ,MOV(37,@89d45884@[3]) ,MOV(0,@89d45884@[4]) ,MOV(1,@89d45884@[5]) ,MOV(1,@89d45884@[6]) ,MOV(0,@89d45884@[7]) ,MOV(0,@89d45884@[8]) ,MOV(@73ebb0c9@.Mailbox.InitiateConnection.Out.C_REF,@89d45884@[9]) ,SWPB(@73ebb0c9@.Mailbox.InitiateConnection.Out.SlaveAddress,REVERSE,@73ebb0c9@.Util.ByteSwapUtil) ,MOV(@73ebb0c9@.Util.ByteSwapUtil,@89d45884@[10]) ] ,XIC(@73ebb0c9@.MailboxCommand.AbortConnection) [MOV(100,@73ebb0c9@.BP.LastWrite) ,MOV(11,@89d45884@[1]) ,MOV(16386,@89d45884@[2]) ,MOV(38,@89d45884@[3]) ,MOV(0,@89d45884@[4]) ,MOV(1,@89d45884@[5]) ,MOV(1,@89d45884@[6]) ,MOV(0,@89d45884@[7]) ,MOV(0,@89d45884@[8]) ,MOV(@73ebb0c9@.Mailbox.InitiateConnection.Out.C_REF,@89d45884@[9]) ,COP(@73ebb0c9@.Mailbox.AbortConnection.Out.ReasonCode,@89d45884@[10],1) ] ,XIC(@73ebb0c9@.MailboxCommand.Class2AcyclicRead) [MOV(100,@73ebb0c9@.BP.LastWrite) ,MOV(12,@89d45884@[1]) ,MOV(16386,@89d45884@[2]) ,MOV(39,@89d45884@[3]) ,MOV(0,@89d45884@[4]) ,MOV(1,@89d45884@[5]) ,MOV(1,@89d45884@[6]) ,MOV(0,@89d45884@[7]) ,MOV(0,@89d45884@[8]) ,MOV(@73ebb0c9@.Mailbox.Class2AcyclicRead.Out.C_REF,@89d45884@[9]) ,COP(@73ebb0c9@.Mailbox.Class2AcyclicRead.Out.Index,@89d45884@[10],1) ,SWPB(@73ebb0c9@.Mailbox.Class2AcyclicRead.Out.Length,REVERSE,@73ebb0c9@.Util.ByteSwapUtil) ,MOV(@73ebb0c9@.Util.ByteSwapUtil,@89d45884@[11]) ] ,XIC(@73ebb0c9@.MailboxCommand.Class2AcyclicWrite) [MOV(100,@73ebb0c9@.BP.LastWrite) ,MOV(13,@89d45884@[1]) ,MOV(16386,@89d45884@[2]) ,MOV(40,@89d45884@[3]) ,MOV(@73ebb0c9@.Mailbox.Class2AcyclicWrite.Out.DataSize,@89d45884@[4]) ,MOV(@73ebb0c9@.Mailbox.Class2AcyclicWrite.Out.DataSize,@73ebb0c9@.Mailbox.Class2AcyclicWrite.Out.Length) ,MOV(1,@89d45884@[5]) ,MOV(1,@89d45884@[6]) ,MOV(0,@89d45884@[7]) ,MOV(0,@89d45884@[8]) ,MOV(@73ebb0c9@.Mailbox.Class2AcyclicWrite.Out.C_REF,@89d45884@[9]) ,COP(@73ebb0c9@.Mailbox.Class2AcyclicWrite.Out.Index,@89d45884@[10],1) ,SWPB(@73ebb0c9@.Mailbox.Class2AcyclicWrite.Out.Length,REVERSE,@73ebb0c9@.Util.ByteSwapUtil) ,MOV(@73ebb0c9@.Util.ByteSwapUtil,@89d45884@[11]) ,COP(@73ebb0c9@.Mailbox.Class2AcyclicWrite.Out.Data[0],@89d45884@[17],200) ] ,XIC(@73ebb0c9@.MailboxCommand.SynchCRC) [MOV(@73ebb0c9@.CRC.In.ProfibusCRC,@73ebb0c9@.CRC.Out.ProfibusCRC) ,MOV(@73ebb0c9@.CRC.In.ModuleCRC,@73ebb0c9@.CRC.Out.ModuleCRC) ,OTU(@73ebb0c9@.MailboxCommand.SynchCRC) ] ] ,LIM(1,@73ebb0c9@.BP.LastWrite,4) [CPT(@73ebb0c9@.BP.BlockIndex,(@73ebb0c9@.BP.LastWrite-1)*400) ,LIM(1,@73ebb0c9@.BP.LastWrite,3) COP(@73ebb0c9@.Output[@73ebb0c9@.BP.BlockIndex],@89d45884@[1],200) ,EQU(@73ebb0c9@.BP.LastWrite,4) COP(@73ebb0c9@.Output[1200],@89d45884@[1],168) ,COP(@73ebb0c9@.MailboxControl.Out_Last_Out_MB,@89d45884@[201],2) ,COP(@73ebb0c9@.CRC.Out.ProfibusCRC,@89d45884@[204],4) ] ,MOV(@73ebb0c9@.BP.LastWrite,@89d45884@[0]) ];
END_ROUTINE
END_ADD_ON_INSTRUCTION

VAR_GLOBAL   (* controller tags *)
   MVI69PDPMV1 : PDPMV1_ModuleDef;
   Local:1:O : AB:1769_MODULE_INT_482Bytes:O:0;
   AOI69PDPMV1_240 : AOI69PDPMV1_240;
   Local:1:I : AB:1769_MODULE_INT_488Bytes:I:0;
END_VAR

PROGRAM MainProgram

ROUTINE MainRoutine   (* ladder *)
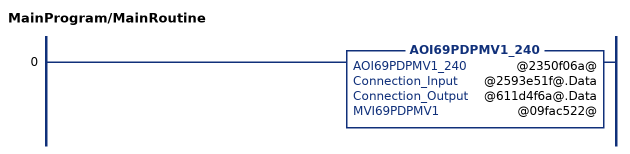
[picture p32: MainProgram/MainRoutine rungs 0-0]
   0: AOI69PDPMV1_240(@2350f06a@,@2593e51f@.Data,@611d4f6a@.Data,@09fac522@);
END_ROUTINE
END_PROGRAM
